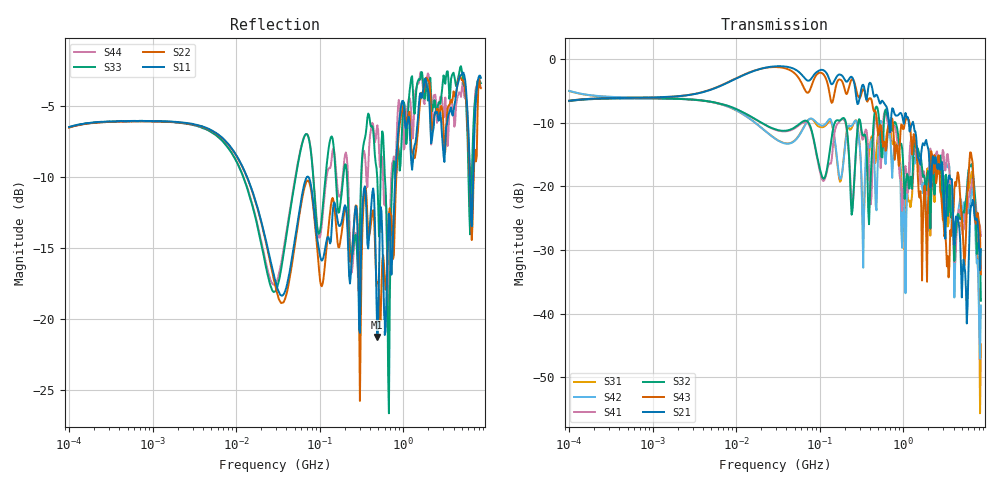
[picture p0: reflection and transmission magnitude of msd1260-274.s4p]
# MHz S MA R 50
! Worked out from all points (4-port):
!   498 points, 100 kHz to 8.5 GHz, reference 50 ohm
!   strongest paths, dB at 100 kHz, 1.698 MHz, 29.49 MHz, 500.7 MHz, 8.5 GHz:
!     S21: -6.6, -5.9, -1.2, -6.1, -29.9
!     S43: -6.6, -5.9, -1.3, -12.0, -33.8
!     S32: -6.6, -6.3, -11.1, -8.2, -38.0
!     S41: -6.6, -6.3, -11.1, -10.5, -27.8
!     S42: -5.0, -6.2, -12.6, -14.5, -38.7
!     S31: -5.0, -6.2, -12.5, -11.5, -44.8
!   lowest |S11| = -21.3 dB at 489.4 MHz (marker M1), VSWR 1.19, Z = 54.7 - j7.75 ohm
!   |S11| at or under -10 dB: 13.49 MHz to 70.21 MHz (56.72 MHz wide, 136 % of centre); 73.2 MHz to 803.2 MHz (730 MHz wide, 167 % of centre); 6.28 GHz to 6.881 GHz (600.4 MHz wide, 9.12 % of centre)
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0.1  0.4744 16.8  0.4693 17.9  0.5597 -15.0  0.4674 -163.0
     0.4693 17.9  0.4723 17.0  0.4667 -163.0  0.5614 -15.1
     0.5597 -15.0  0.4667 -163.0  0.4739 16.9  0.4695 17.9
     0.4674 -163.0  0.5614 -15.1  0.4695 17.9  0.473 17.0
489.3566  0.0862 -54.7  0.5127 -87.8  0.2305 -4.0  0.3324 -35.0
          0.5127 -87.8  0.1334 -51.8  0.4152 -30.2  0.1164 21.9
          0.2305 -4.0  0.4152 -30.2  0.3121 -71.1  0.2906 -112.6
          0.3324 -35.0  0.1164 21.9  0.2906 -112.6  0.4815 -50.2
1970.81  0.6448 -171.2  0.2024 103.5  0.1385 152.9  0.09223 -173.1
         0.2024 103.5  0.6917 -166.6  0.1318 155.0  0.0448 -177.0
         0.1385 152.9  0.1318 155.0  0.5881 -168.1  0.0681 -131.8
         0.09223 -173.1  0.0448 -177.0  0.0681 -131.8  0.7338 -172.2
3041.538  0.3745 81.5  0.09595 -75.1  0.07717 37.5  0.1839 40.3
          0.09595 -75.1  0.4661 73.8  0.05435 46.1  0.1577 45.1
          0.07717 37.5  0.05435 46.1  0.722 82.4  0.05227 -84.1
          0.1839 40.3  0.1577 45.1  0.05227 -84.1  0.5123 64.9
4913.36  0.7233 -90.4  0.02331 57.1  0.04874 -104.8  0.05894 -107.0
         0.02331 57.1  0.706 -98.0  0.05613 -78.8  0.07848 -117.1
         0.04874 -104.8  0.05613 -78.8  0.7778 -95.3  0.0667 84.5
         0.05894 -107.0  0.07848 -117.1  0.0667 84.5  0.6057 -90.3
6611.76  0.2117 89.5  0.07054 48.0  0.1302 63.6  0.1045 97.9
         0.07054 48.0  0.1894 100.7  0.1495 78.2  0.0987 56.2
         0.1302 63.6  0.1495 78.2  0.302 73.4  0.167 -46.6
         0.1045 97.9  0.0987 56.2  0.167 -46.6  0.3289 96.3
8500  0.707 -54.1  0.03204 -79.7  0.005764 -55.9  0.04082 -141.7
      0.03204 -79.7  0.6506 -40.7  0.01262 -141.2  0.01159 -94.9
      0.005764 -55.9  0.01262 -141.2  0.6772 -53.7  0.02039 -70.4
      0.04082 -141.7  0.01159 -94.9  0.02039 -70.4  0.6566 -53.1
